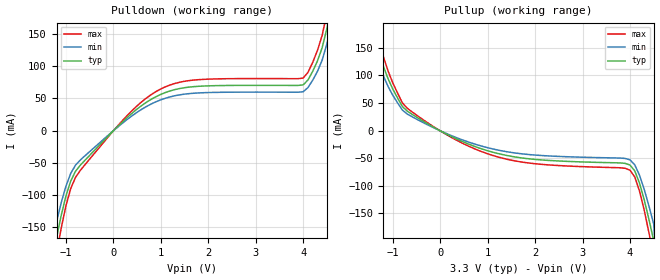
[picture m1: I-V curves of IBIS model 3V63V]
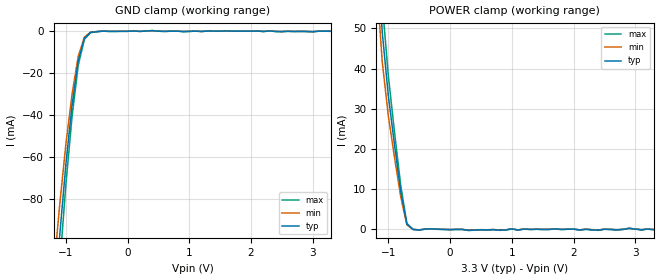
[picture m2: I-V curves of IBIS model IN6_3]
[IBIS Ver]   2.1
[File name]   ics551_3.ibs
[File Rev]   2.0
[Date]   05/16/2000
[Source]   ICS MicroClock Applications Engineering 2
[Disclaimer] This information is for modeling purposes only, and is
(C) Copyright Integrated Circuit Systems, Inc. 1997-2001
   All rights reserved
ICS hereby grants the user of this IBIS model a non-exclusive,
nontransferable license to use this IBIS model under the following terms.
Before using this IBIS model, the user should read this license.
If the user does not accept these terms,  the IBIS model should be
returned to ICS within 30 days.
   The user is granted this license only to use the IBIS model and
is not granted rights to sell, load, rent, lease or license the IBIS
model in whole or in part, or in modified form to anyone other than
user. User may modify the IBIS model to suit its specific
applications but rights to derivative works and such modifications
shall belong to ICS.
   This IBIS model is provided on an "AS IS" basis and ICS makes
absolutely no warranty with respect to the information contained
herein. ICS DISCLAIMS AND CUSTOMER WAIVES ALL WARRANTIES, EXPRESS
OR IMPLIED, INCLUDING WARRANTIES OF MERCHANTABILITY OR FITNESS FOR
A PARTICULAR PURPOSE. The entire risk as to quality and performance
is with the Customer. ACCORDINGLY, IN NO EVENT SHALL THE COMPANY BE
LIABLE FOR ANY DAMAGES, WHETHER IN CONTRACT OR TORT,INCLUDING ANY
LOST PROFITS OR OTHER INCIDENTAL, CONSEQUENTIAL, EXEMPLARY, OR
PUNITIVE DAMAGES ARISING OUT OF THE USE OR APPLICATION OF THE IBIS
model provided in this package. Further, ICS reserves the right to
make changes without notice to any product herein to improve
reliability, function, or design. ICS does not convey any license
under patent rights or any other intellectual property rights,
including those of third parties.
   ICS is not obligated to provide maintenance or support
for the licensed IBIS model.
[Component]   ICS551
[Manufacturer] Integrated Circuit Systems Inc.
[Package]
|   typ   min   max
R_pkg   40m   35m   45m
L_pkg   1.65nH   1.35nH   1.95nH
C_pkg   0.24pF   0.14pF   0.34pF
[pin]   signal_name   model_name   R_pin   L_pin   C_pin
   1   ICLK   IN6_3
   2   Q1   3V63V
   3   Q2   3V63V
   4   Q3   3V63V
   5   Q4   3V63V
| Models and submodels in the file (2): 3V63V (Output), IN6_3 (Input)
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|   ICS551 3.3V Clock Drive Model
| This model is suitable for all output pins on the
| ICS551
[Model]   3V63V
Model_type   Output
Polarity   Non-Inverting
|   typ   min   max
C_comp   5pF   4pF   6pF
|   typ   min   max
[Voltage range]  3.3V   3.15V   3.45V
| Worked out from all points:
|   slope of the pulldown table from 0 to 0.495 V, typ, clamps not added: 14.9 ohm
|   slope of the pullup table from 0 to 0.495 V, typ, clamps not added: 24.2 ohm
[pulldown]
|Voltage I (typ)   I (min)   I (max)
-3.3V     -3A        -3A        -3A
-1.3V     -199.9mA   -169.9mA   -229.9mA
-1.2V     -166.1mA   -141.2mA   -191mA
-1.1V     -131mA     -111.3mA   -150.6mA
-800mV    -63.14mA   -53.66mA   -72.61mA
400mV     27.29mA    23.2mA     31.39mA
1.1V      58.96mA    50.11mA    67.8mA
4V        70.65mA    60.05mA    81.25mA
4.3V      107.5mA    91.34mA    123.6mA
4.5V      157.8mA    134.1mA    181.5mA
4.6V      195.8mA    166.4mA    225.2mA
6.6V      3A         3A         3A
[pullup]
|Voltage I (typ)   I (min)   I (max)
-3.3V     3A         3A         3A
-1.4V     190.5mA    161.9mA    219.1mA
-1.3V     149.2mA    126.8mA    171.6mA
-1.2V     116.4mA    98.91mA    133.8mA
-800mV    43.62mA    37.08mA    50.17mA
400mV     -17.51mA   -14.88mA   -20.14mA
1.6V      -48.26mA   -41.02mA   -55.49mA
4V        -62.64mA   -53.25mA   -72.04mA
4.2V      -95.46mA   -81.14mA   -109.8mA
4.4V      -161.7mA   -137.4mA   -185.9mA
4.5V      -199.9mA   -169.9mA   -229.9mA
6.6V      -3A        -3A        -3A
[Ramp]
|   typ   min   max
dV/dt_r   1.31/0.41n   1.24/0.45n   1.37/0.37n
dV/dt_f   1.54/0.34n   1.46/0.38n   1.62/0.31n
|   3.3V  INPUT  Model
| This model is suitable for ALL INPUT Pin
[Model]   IN6_3
Model_type   Input
Polarity   Non-Inverting
Vinl = 1.15V   | input logic "low" DC voltage
Vinh = 2.15V   | input logic "high" DC voltage
Vmeas = 1.65V
|   typ   min   max
C_comp   5pF   4pF   6pF
|   typ   min   max
[Voltage range]  3.3V   2.97V   3.63V
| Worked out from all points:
|   GND clamp passes 1 mA (typ) near -0.61 V on its own axis
[GND_clamp]
|Voltage I (typ)   I (min)   I (max)
-3.3V     -3A        -3A        -3A
-1.2V     -135.8mA   -115.4mA   -156.1mA
-1.1V     -97.7mA    -83.05mA   -112.4mA
-1V       -63.72mA   -54.16mA   -73.28mA
-900mV    -35.55mA   -30.22mA   -40.89mA
-800mV    -14.29mA   -12.15mA   -16.44mA
-700mV    -3.48mA    -2.958mA   -4.002mA
-600mV    -708uA     -601.8uA   -814.2uA
-400mV    -72.3uA    -61.47uA   -83.16uA
400mV     155uA      131.8uA    178.2uA
900mV     -299uA     -254.2uA   -343.8uA
3.3V      -163uA     -138.6uA   -187.5uA
[POWER_clamp]
|Voltage I (typ)   I (min)   I (max)
-3.3V     3A         3A         3A
-1.2V     75.3mA     64.01mA    86.6mA
-1.1V     49.18mA    41.8mA     56.56mA
-1V       33.09mA    28.13mA    38.06mA
-900mV    20.92mA    17.78mA    24.06mA
-800mV    9.423mA    8.01mA     10.84mA
-700mV    1.2mA      1.02mA     1.38mA
-600mV    -118uA     -100.3uA   -135.7uA
1.7V      18.6uA     15.77uA    21.34uA
2.4V      -299uA     -254.2uA   -343.8uA
2.9V      155uA      131.8uA    178.2uA
3.3V      -163uA     -138.6uA   -187.5uA
